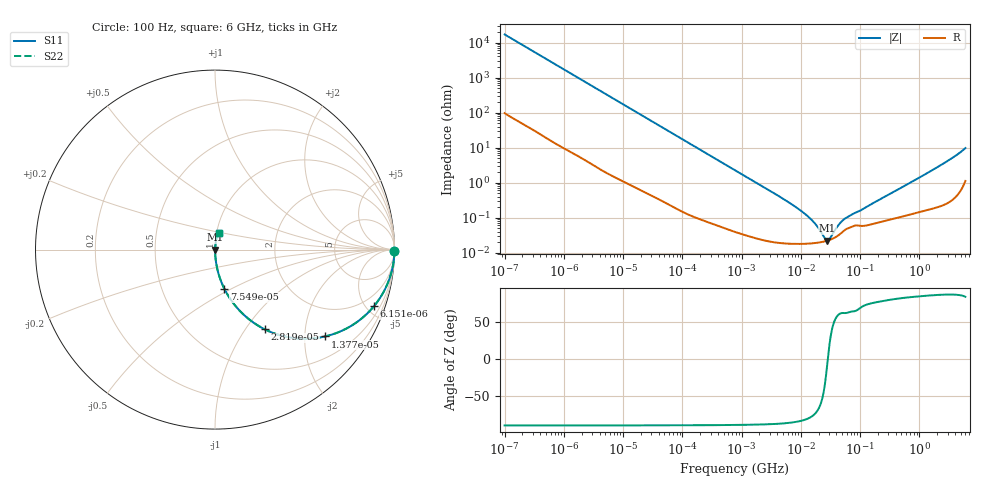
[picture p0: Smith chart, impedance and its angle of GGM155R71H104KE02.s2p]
!Murata Part Number: GGM155R71H104KE02
!These Parameters are Measured in Series Mode Connection
!Data Generated on Jun 19, 2026
!  o--ll--o
!Port1  Port2
!  o------o
!Operation Temp=25[degC], DC Bias Voltage=0[V]
!Freq. Start=100[Hz] Stop=6[GHz] 401[Steps]
# Hz S RI R 50
!Freq.(Hz) S11(Real) S11(Imag) S21(Real) S21(Imag) S12(Real) S12(Imag) S22(Real) S22(Imag)
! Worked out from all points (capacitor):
!   401 points, 100 Hz to 6 GHz, reference 50 ohm
!   read as one part in series: C = 93.4 nF near 109 Hz
!   lowest |Z| = 22.1 mohm at 27.84 MHz (marker M1)
!   series resonance near 28.59 MHz, so ESL is about 330 pH
!   S11 on the Smith chart (normalised r, x): 100 Hz: open; 6.151 kHz: 1.03, -5.61; 13.77 kHz: 1.02, -2.51; 28.19 kHz: 1.01, -1.23; 75.5 kHz: 1.00, -0.46; 6 GHz: 1.02, +0.19
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100  0.9999 -0.00587  6.78e-05 0.00587  6.78e-05 0.00587  0.9999 -0.00587
627  0.9985 -0.0365  0.00154 0.0365  0.00154 0.0365  0.9985 -0.0365
2008  0.9859 -0.115  0.0141 0.115  0.0141 0.115  0.9859 -0.115
6151  0.886 -0.315  0.114 0.315  0.114 0.315  0.886 -0.315
9204  0.7778 -0.4127  0.2222 0.4127  0.2222 0.4127  0.7778 -0.4127
13772  0.6119 -0.484  0.3881 0.484  0.3881 0.484  0.6119 -0.484
28191  0.2767 -0.4437  0.7233 0.4437  0.7233 0.4437  0.2767 -0.4437
40335  0.1588 -0.3617  0.8412 0.3617  0.8412 0.3617  0.1588 -0.3617
75495  0.0523 -0.2187  0.9477 0.2187  0.9477 0.2187  0.0523 -0.2187
202169  0.00833 -0.0859  0.9917 0.0859  0.9917 0.0859  0.00833 -0.0859
774597  0.000909 -0.0228  0.9991 0.0228  0.9991 0.0228  0.000909 -0.0228
6644369  0.000186 -0.00255  0.9998 0.00255  0.9998 0.00255  0.000186 -0.00255
1.555665e7  0.000185 -0.000809  0.9998 0.000809  0.9998 0.000809  0.000185 -0.000809
1.946e7  0.000193 -0.000493  0.9998 0.000493  0.9998 0.000493  0.000193 -0.000493
2.545746e7  0.00021 -0.000146  0.9998 0.000146  0.9998 0.000146  0.00021 -0.000146
2.784235e7  0.000219 -3.31e-05  0.9998 3.31e-05  0.9998 3.31e-05  0.000219 -3.31e-05
3.045065e7  0.00023 7.9e-05  0.9998 -7.9e-05  0.9998 -7.9e-05  0.00023 7.9e-05
4.35672e7  0.000316 0.000538  0.9997 -0.000538  0.9997 -0.000538  0.000316 0.000538
5.449875e7  0.000436 0.000804  0.9996 -0.000804  0.9996 -0.000804  0.000436 0.000804
3.124326e8  0.000889 0.00457  0.9991 -0.00457  0.9991 -0.00457  0.000889 0.00457
2.142435e9  0.00288 0.0291  0.9971 -0.0291  0.9971 -0.0291  0.00288 0.0291
6e9  0.0199 0.0935  0.9801 -0.0935  0.9801 -0.0935  0.0199 0.0935
